PROGRAM P_IEC61850MAIN
VAR
END_VAR

IF NOT fbIEDCriticalSection.Enter() THEN
	RETURN;
END_IF

fbIEDServer.Execute();
fbIEDServerSession1();

(*
fbIEDServerSession2();
...
fbIEDServerSessionN();
*)

fbIEDCriticalSection.Leave();

END_PROGRAM
